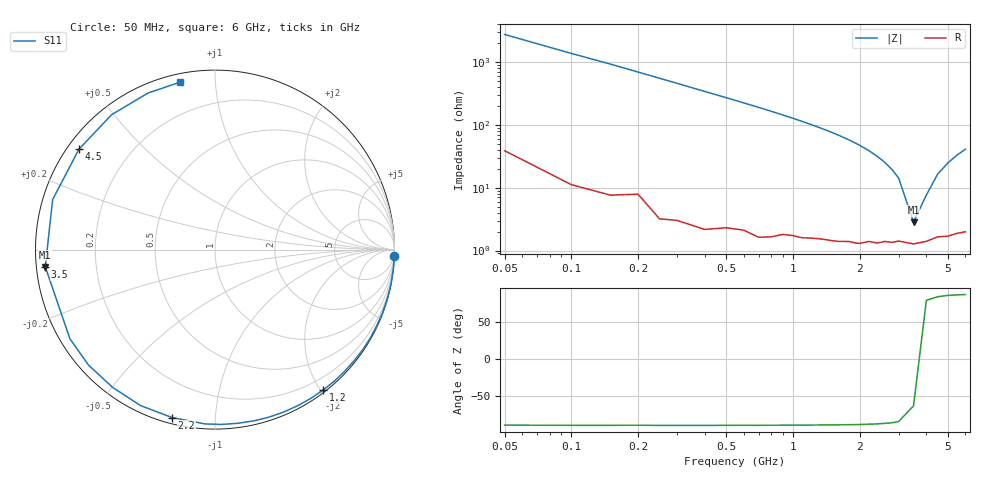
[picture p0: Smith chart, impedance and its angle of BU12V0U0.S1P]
! Infineon Technologies  Discrete & RF Semiconductors
! BB 833
! Si Tuning Diode in SOD323
! VR = 12 V
! S-Parameters:  June  1999
# GHz  S  MA  R  50
!  f  S11
! GHz  MAG  ANG
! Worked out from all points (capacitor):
!   34 points, 50 MHz to 6 GHz, reference 50 ohm
!   read as one part to ground: C = 1.17 pF near 50 MHz
!   lowest |Z| = 2.83 ohm at 3.5 GHz (marker M1)
!   series resonance near 3.626 GHz, so ESL is about 1.7 nH
!   S11 on the Smith chart (normalised r, x): 50 MHz: 1, -55; 1.2 GHz: 0.03, -2.04; 2.2 GHz: 0.03, -0.78; 3.5 GHz: 0.03, -0.05; 4.5 GHz: 0.03, +0.33; 6 GHz: 0.04, +0.81
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0.05  0.9995 -2.1
0.25  0.999 -10.4
0.4  0.9981 -16.8
0.6  0.996 -25.3
0.7  0.9958 -29.6
0.8  0.9943 -34.0
1  0.9907 -43.0
1.1  0.9896 -47.6
1.2  0.9878 -52.3
1.3  0.9859 -57.2
1.4  0.9842 -62.0
1.5  0.9826 -67.0
1.6  0.9808 -72.1
1.7  0.9784 -77.3
1.8  0.976 -82.6
1.9  0.9747 -87.9
2  0.9729 -93.3
2.2  0.9658 -104.3
2.4  0.963 -115.5
2.6  0.9564 -126.5
2.8  0.9542 -137.6
3  0.9488 -148.4
3.5  0.9504 -174.2
4  0.9466 162.9
4.5  0.942 143.6
5  0.9469 127.5
5.5  0.9488 113.2
6  0.9532 101.7
